FUNCTION_BLOCK FB_DO_IED_LD1_ATCC1_BndCtrChg EXTENDS FB_AcsiCommonControllableDataClass
VAR_INPUT
	mxVal: FB_AcsiDATypeAnalogueValue := (fc:=ACSI_FC_MX, TrgOp:=ACSI_TrgOp_dchg, bLinkResult:=THIS^.AddDataToContainer(ipData:=mxVal));
	q: FB_AcsiDATypeQuality := (fc:=ACSI_FC_MX, TrgOp:=ACSI_TrgOp_qchg, bLinkResult:=THIS^.AddDataToContainer(ipData:=q));
	t: FB_AcsiDATypeTimeStamp := (fc:=ACSI_FC_MX, bLinkResult:=THIS^.AddDataToContainer(ipData:=t));
	stSeld: FB_AcsiBATypeBOOLEAN := (fc:=ACSI_FC_MX, TrgOp:=ACSI_TrgOp_dchg, bLinkResult:=THIS^.AddDataToContainer(ipData:=stSeld));
	persistent_: FB_AcsiBATypeBOOLEAN := (sObjectName:='persistent', fc:=ACSI_FC_CF, TrgOp:=ACSI_TrgOp_dchg, bLinkResult:=THIS^.AddDataToContainer(ipData:=persistent_));
	ctlModel: FB_AcsiDATypeCtlModels := (fc:=ACSI_FC_CF, TrgOp:=ACSI_TrgOp_dchg, eValue:=E_AcsiCtlModels.DirectWithEnhancedSecurity, bLinkResult:=THIS^.AddDataToContainer(ipData:=ctlModel));
	Oper: FB_AcsiCDC_Oper_CODEDENUM := (fc:=ACSI_FC_CO, bLinkResult:=THIS^.AddDataToContainer(ipData:=Oper));
	
	fbControl: FB_DirectControl := (ipCtrl:=THIS^.AddServerJob(ipEvent:=fbControl, ipCompletion:=fbControl), eType:=E_AcsiCDCType.BAC, ipBehVal:=fbIED.IEDLD1.ATCC1.Beh.stVal);
END_VAR
VAR
END_VAR

END_FUNCTION_BLOCK
